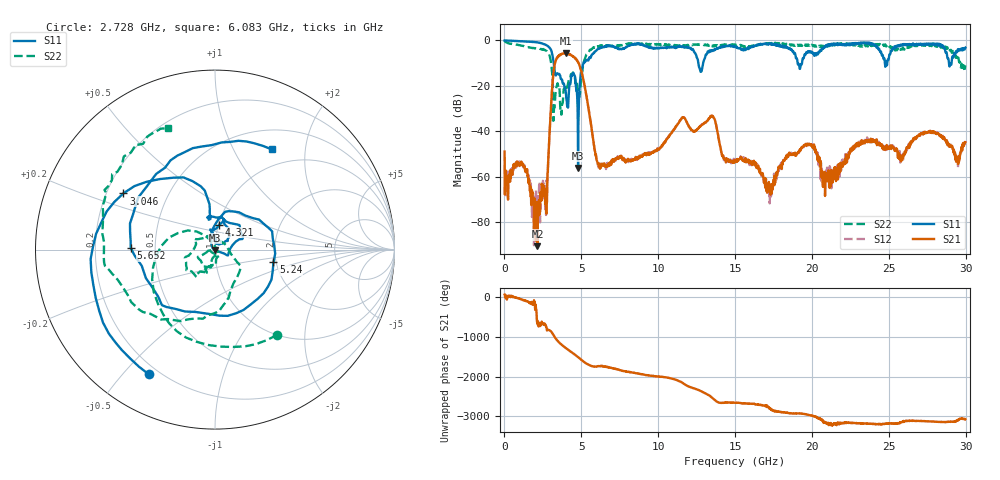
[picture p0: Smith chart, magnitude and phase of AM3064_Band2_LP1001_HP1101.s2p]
# Hz S DB R 50.0
!freq dBS11 angS11 dBS21 angS21 dBS12 angS12 dBS22 angS22
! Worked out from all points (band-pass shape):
!   1600 points, 10 MHz to 29.98 GHz, reference 50 ohm
!   highest |S21| = -5.61 dB at 4.002 GHz (marker M1); lowest = -90.4 dB at 2.147 GHz (marker M2)
!   |S21| within 3 dB of the highest: 3.354 GHz to 4.693 GHz (1.34 GHz wide, 33.3 % of centre)
!   lowest |S11| = -56.0 dB at 4.79 GHz (marker M3), VSWR 1.00, Z = 50 - j0.15 ohm
!   |S11| at or under -10 dB: 3.204 GHz to 5.138 GHz (1.933 GHz wide, 46.4 % of centre); 12.61 GHz to 12.92 GHz (312.3 MHz wide, 2.45 % of centre); 19.07 GHz to 19.35 GHz (284 MHz wide, 1.48 % of centre)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
!   |S22| runs from -35.3 to -0.2 dB; largest |S21 - S12| = 0.019
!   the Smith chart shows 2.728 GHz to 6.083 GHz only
!   S11 on the Smith chart (normalised r, x): 2.728 GHz: 0.16, -0.59; 3.046 GHz: 0.27, +0.26; 4.321 GHz: 1.01, +0.29; 5.24 GHz: 1.93, -0.31; 5.652 GHz: 0.36, +0.01; 6.083 GHz: 0.75, +1.43
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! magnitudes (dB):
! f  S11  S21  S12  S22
! 10 MHz  0.0  -48.9  -54.8  -0.2
! 1.191 GHz  -0.4  -54.3  -54.6  -2.4
! 2.147 GHz  -0.9  -90.4  -67.5  -3.6
! 2.728 GHz  -2.1  -76.1  -70.4  -4.6
! 3.046 GHz  -4.5  -26.9  -26.9  -10.5
! 3.346 GHz  -15.4  -8.8  -8.8  -21.5
! 4.002 GHz  -23.4  -5.6  -5.7  -20.6
! 4.321 GHz  -17.0  -6.5  -6.4  -15.0
! 4.79 GHz  -56.0  -9.5  -9.5  -21.4
! 5.015 GHz  -12.9  -13.9  -13.9  -15.1
! 5.24 GHz  -9.5  -21.0  -20.9  -8.0
! 5.652 GHz  -6.6  -37.8  -37.8  -4.0
! 6.083 GHz  -3.9  -54.3  -54.4  -2.8
! 10 GHz  -3.4  -47.8  -47.8  -1.8
! 12.77 GHz  -13.8  -37.5  -37.3  -1.9
! 13.49 GHz  -4.4  -33.2  -33.2  -2.3
! 15 GHz  -2.7  -53.2  -53.7  -1.8
! 17.25 GHz  -1.5  -66.6  -71.6  -1.2
! 19.99 GHz  -5.1  -46.1  -46.0  -1.9
! 20.83 GHz  -3.1  -57.9  -58.4  -2.4
! 25 GHz  -8.2  -47.6  -46.6  -2.3
! 29.98 GHz  -3.2  -44.7  -46.1  -10.9
